(* Logix 5000 AddOnInstructionDefinition export G500ETH_Generic_Default_IO; software revision 20.01 *)

ADD_ON_INSTRUCTION G500ETH_Generic_Default_IO   (* revision 1.0 *)
// Simple interface for generic default IO mapping that uses Input Assembly Instance 150 and Output Assembly Instance 100.
VAR_IN_OUT
   I_Data : INT[3]; {required}   // Input data
   O_Data : INT[2]; {required}   // Output data
        [0]   // Output
END_VAR
VAR_INPUT
   Start : BOOL; {access Read Only, required}   // Start/Stop
   Direction : BOOL; {access Read Only, required}   // Forward (0) / Reverse (1)
   Jog : BOOL; {access Read Only, required}   // Jog enable
   CoastStop : BOOL; {access Read Only, required}   // Coast to stop
   EStop : BOOL; {access Read Only, required}   // Emergency stop
   Reset : BOOL; {access Read Only, required}   // Reset fault condition on a positive edge
   Heartbeat : BOOL; {access Read Only, required}   // Heartbeat command
   FrequencyCommand : INT; {access Read Only, required}   // Frequency command
END_VAR
VAR_OUTPUT
   Running : BOOL; {access Read Only, visible}   // Running/Stopped
   RunningDir : BOOL; {access Read Only, visible}   // Running direction forward (0) /reverse (1)
   Faulted : BOOL; {access Read Only, visible}   // Faults present
   HeartbeatFeedback : BOOL; {access Read Only, visible}   // Heartbeat feedback
   OutputFrequency : INT; {access Read Only, visible}   // Output frequency
END_VAR

ROUTINE Logic   (* ladder *)
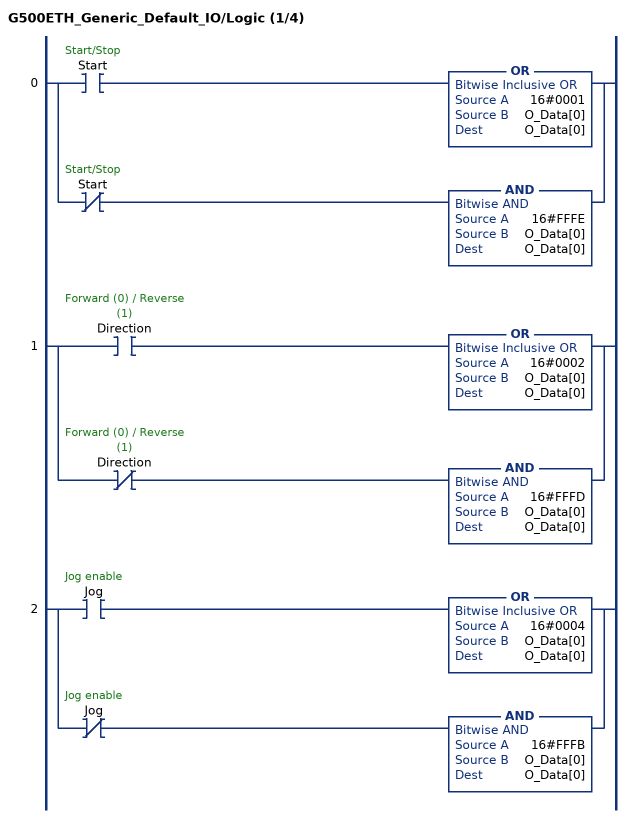
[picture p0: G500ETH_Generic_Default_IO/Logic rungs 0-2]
   0: [XIC(Start) OR(16#0001,O_Data[0],O_Data[0]) ,XIO(Start) AND(16#FFFE,O_Data[0],O_Data[0]) ];
   1: [XIC(Direction) OR(16#0002,O_Data[0],O_Data[0]) ,XIO(Direction) AND(16#FFFD,O_Data[0],O_Data[0]) ];
   2: [XIC(Jog) OR(16#0004,O_Data[0],O_Data[0]) ,XIO(Jog) AND(16#FFFB,O_Data[0],O_Data[0]) ];
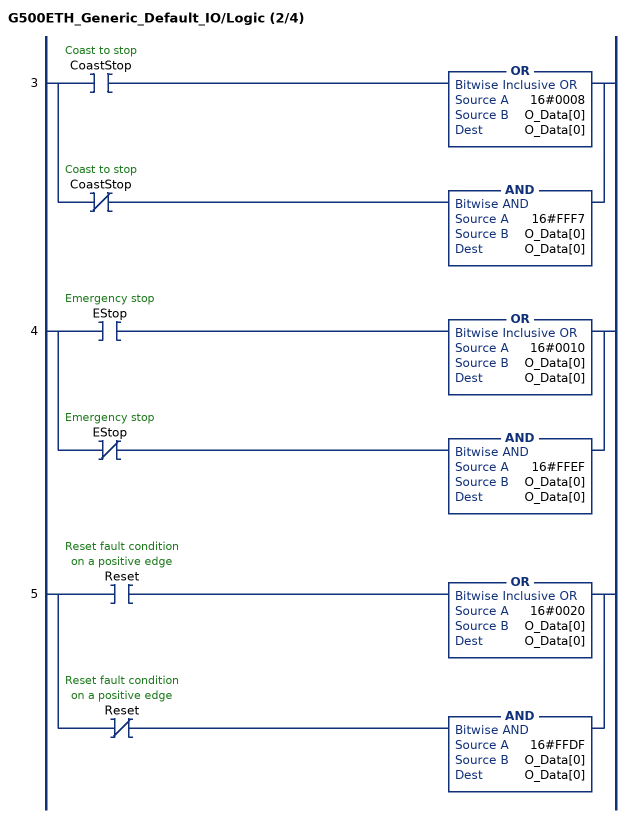
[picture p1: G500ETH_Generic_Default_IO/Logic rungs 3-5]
   3: [XIC(CoastStop) OR(16#0008,O_Data[0],O_Data[0]) ,XIO(CoastStop) AND(16#FFF7,O_Data[0],O_Data[0]) ];
   4: [XIC(EStop) OR(16#0010,O_Data[0],O_Data[0]) ,XIO(EStop) AND(16#FFEF,O_Data[0],O_Data[0]) ];
   5: [XIC(Reset) OR(16#0020,O_Data[0],O_Data[0]) ,XIO(Reset) AND(16#FFDF,O_Data[0],O_Data[0]) ];
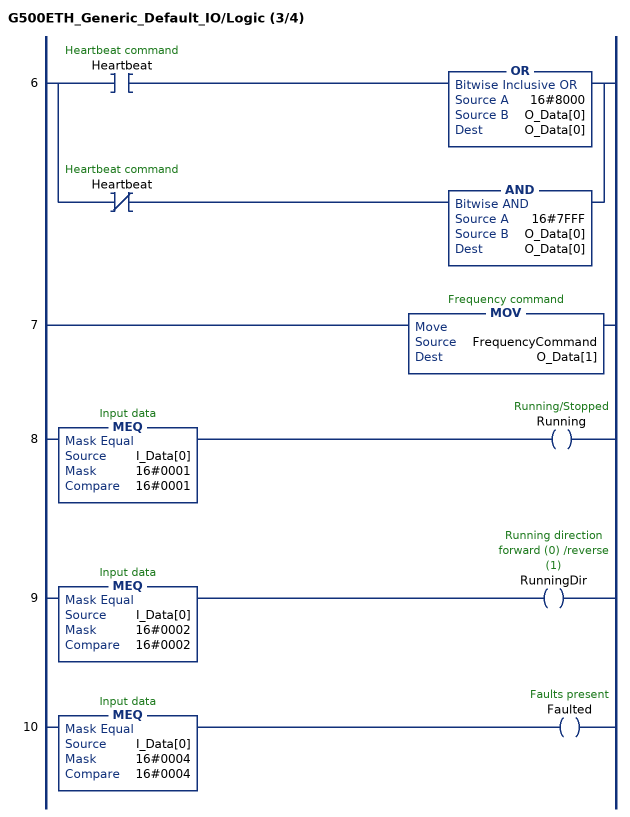
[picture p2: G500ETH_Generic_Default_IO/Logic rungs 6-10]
   6: [XIC(Heartbeat) OR(16#8000,O_Data[0],O_Data[0]) ,XIO(Heartbeat) AND(16#7FFF,O_Data[0],O_Data[0]) ];
   7: MOV(FrequencyCommand,O_Data[1]);
   8: MEQ(I_Data[0],16#0001,16#0001)OTE(Running);
   9: MEQ(I_Data[0],16#0002,16#0002)OTE(RunningDir);
   10: MEQ(I_Data[0],16#0004,16#0004)OTE(Faulted);
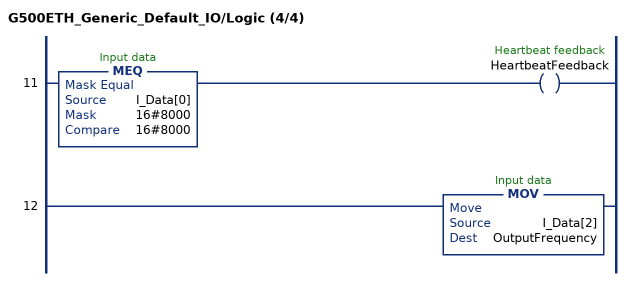
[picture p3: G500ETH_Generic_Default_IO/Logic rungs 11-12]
   11: MEQ(I_Data[0],16#8000,16#8000)OTE(HeartbeatFeedback);
   12: MOV(I_Data[2],OutputFrequency);
END_ROUTINE
END_ADD_ON_INSTRUCTION
